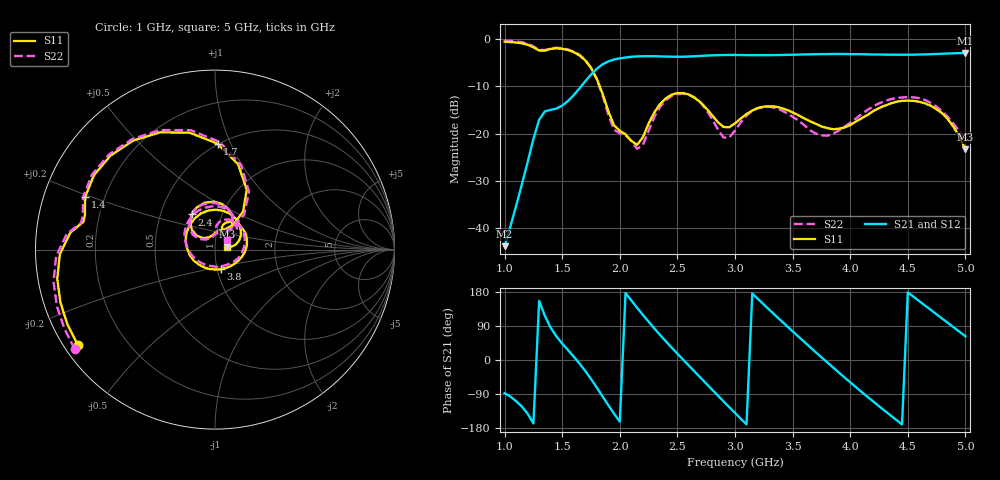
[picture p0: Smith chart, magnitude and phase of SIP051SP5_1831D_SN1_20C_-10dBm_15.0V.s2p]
# GHz  S  dB  R  50
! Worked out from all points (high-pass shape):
!   81 points, 1 GHz to 5 GHz, reference 50 ohm
!   highest |S21| = -3.01 dB at 5 GHz (marker M1); lowest = -43.8 dB at 1 GHz (marker M2)
!   |S21| within 3 dB of the highest: 1.818 GHz to end of sweep
!   lowest |S11| = -23.3 dB at 5 GHz (marker M3), VSWR 1.15, Z = 57.1 + j1.77 ohm
!   |S11| at or under -10 dB: 1.825 GHz to end of sweep
!   |S22| runs from -23.2 to -0.4 dB; largest |S21 - S12| = 0.0018
!   S11 on the Smith chart (normalised r, x): 1 GHz: 0.04, -0.31; 1.4 GHz: 0.13, +0.19; 1.7 GHz: 0.49, +0.89; 2.4 GHz: 0.72, +0.30; 3.8 GHz: 1.04, -0.23; 5 GHz: 1.14, +0.04
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1  -0.63 -145.3  -43.77 -87.6  -43.93 -87.4  -0.37 -144.6
1.3  -2.50 168.1  -17.09 155.9  -17.07 155.8  -2.37 168.7
1.4  -2.15 158.0  -15.01 85.2  -14.98 85.3  -2.03 158.3
1.55  -2.39 126.9  -13.14 26.2  -13.14 26.2  -2.28 126.8
1.7  -4.58 88.6  -8.99 -29.0  -9.01 -28.9  -4.44 87.5
1.85  -11.58 53.5  -5.41 -96.1  -5.42 -96.1  -11.93 50.2
2.05  -20.20 87.0  -3.97 176.8  -3.96 176.8  -20.36 86.1
2.2  -20.82 135.4  -3.70 119.2  -3.69 119.2  -22.46 132.4
2.35  -13.77 132.5  -3.74 65.9  -3.73 66.0  -14.38 138.6
2.4  -12.57 123.6  -3.77 49.1  -3.77 49.0  -12.95 128.7
2.55  -11.46 91.7  -3.80 0.7  -3.79 0.7  -11.63 94.7
2.75  -14.68 57.0  -3.57 -62.1  -3.57 -62.1  -14.95 55.6
2.9  -18.61 60.2  -3.44 -109.0  -3.43 -109.1  -20.85 64.3
3  -17.86 72.7  -3.43 -139.8  -3.42 -139.8  -19.35 87.6
3.2  -14.60 54.3  -3.49 160.8  -3.49 160.8  -14.64 64.3
3.4  -14.60 16.3  -3.44 103.8  -3.43 103.8  -15.07 19.3
3.7  -17.94 -47.5  -3.27 20.8  -3.27 20.8  -20.00 -68.2
3.8  -18.85 -73.9  -3.24 -6.2  -3.24 -6.2  -20.47 -104.5
4.1  -16.76 -169.2  -3.27 -84.5  -3.26 -84.6  -15.88 172.1
4.35  -13.69 123.4  -3.38 -146.1  -3.39 -146.2  -12.76 121.8
4.65  -13.65 56.7  -3.31 143.6  -3.30 143.7  -12.93 67.1
5  -23.31 13.1  -3.01 62.5  -3.01 62.5  -21.18 38.9
